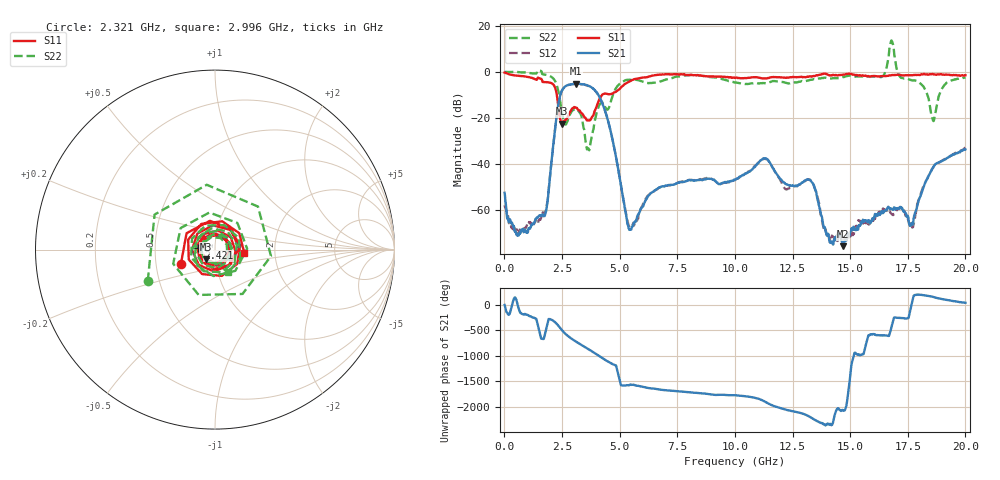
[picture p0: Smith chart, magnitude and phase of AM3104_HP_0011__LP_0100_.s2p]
!Created with skrf (http://scikit-rf.org).
# Hz S RI R 50.0
!freq ReS11 ImS11 ReS21 ImS21 ReS12 ImS12 ReS22 ImS22
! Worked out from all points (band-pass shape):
!   1601 points, 10 MHz to 20 GHz, reference 50 ohm
!   highest |S21| = -5.21 dB at 3.121 GHz (marker M1); lowest = -75.8 dB at 14.69 GHz (marker M2)
!   |S21| within 3 dB of the highest: 2.495 GHz to 3.943 GHz (1.448 GHz wide, 45 % of centre)
!   lowest |S11| = -22.5 dB at 2.509 GHz (marker M3), VSWR 1.16, Z = 44.8 - j4.87 ohm
!   |S11| at or under -10 dB: 2.274 GHz to 4.243 GHz (1.968 GHz wide, 60.4 % of centre)
!   |S22| runs from -34.1 to 13.6 dB; largest |S21 - S12| = 0.03
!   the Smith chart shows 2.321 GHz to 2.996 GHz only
!   S11 on the Smith chart (normalised r, x): 2.321 GHz: 0.67, -0.12; 2.421 GHz: 0.83, +0.02; 2.996 GHz: 1.39, -0.06
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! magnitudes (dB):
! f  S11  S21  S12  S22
! 10 MHz  -0.3  -52.6  -58.0  0.0
! 572.2 MHz  -1.7  -70.9  -70.1  -0.1
! 1.747 GHz  -4.5  -62.7  -61.6  -1.2
! 2.321 GHz  -13.7  -15.3  -15.4  -7.7
! 2.421 GHz  -20.6  -10.3  -10.4  -12.9
! 2.509 GHz  -22.5  -7.9  -8.0  -18.3
! 2.996 GHz  -15.6  -5.3  -5.3  -16.6
! 3.121 GHz  -15.6  -5.2  -5.2  -16.7
! 3.346 GHz  -17.9  -5.3  -5.4  -19.3
! 3.646 GHz  -21.1  -6.1  -6.2  -33.3
! 4.37 GHz  -9.4  -17.1  -17.1  -15.3
! 5.42 GHz  -4.3  -68.7  -67.5  -3.4
! 6.682 GHz  -1.2  -50.5  -50.6  -4.4
! 10.01 GHz  -2.7  -47.0  -47.1  -4.6
! 11.3 GHz  -2.9  -37.6  -37.9  -4.9
! 13.34 GHz  -2.1  -48.0  -48.1  -3.5
! 13.93 GHz  -0.8  -69.0  -69.0  -2.5
! 14.69 GHz  -1.2  -75.8  -71.4  -2.3
! 16.68 GHz  -1.6  -59.1  -60.4  7.2
! 17.69 GHz  -1.6  -66.0  -67.6  -3.7
! 18.6 GHz  -1.1  -41.6  -41.7  -21.3
! 20 GHz  -1.5  -33.7  -33.0  -2.5
